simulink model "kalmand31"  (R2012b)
settings: Solver=ode4  StartTime=0.0  StopTime=10.0  RelTol=1e-3
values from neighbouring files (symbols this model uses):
  ampl = 2    [kalman_d2.m]    (also in kalman_d3.m; kalman_d4.m; diff_filter_1.m = 1)
  fanreg = 0.1    [kalman_d2.m]    (also in kalman_d3.m; kalman_d4.m)
  Kest = kalman(P,1,0.01),    [LQG_1.m]    (also in ss_zwei_eing_1.m = kalman(sys2, Q, R))
  my_sys11 = ss(my_sys11.a,my_sys11.b,eye(2,2),[0;0])    [kalman_d2.m]    (also in kalman_d3.m = ss(my_sys3.a, my_sys3.b(:,1), eye(2,2), 0); kalman_pegel_1.m = c2d(my_sys1,Ts,'zoh'))
  my_sys3 = c2d(my_sys2, Ts, 'zoh')    [kalman_d2.m]    (also in kalman_d3.m)
  Ts = 0.001    [fuellstnd_3.m]    (also in fuellstnd_31.m; kalman_d1.m = 0.05; kalman_d2.m = 0.1; kalman_d3.m = 0.1)
  vnd = 1e-4    (= 0.0001)    [kalman_1.m]    (also in kalman_10.m; kalman_11.m; kalman_12.m; kalman_13.m = 0.01)
  vny = 1e-6    (= 1e-06)    [kalman_1.m]    (also in kalman_10.m; kalman_11.m = ', num2str(vny),' )']); kalman_12.m = ', num2str(vny),' )']); kalman_13.m = ', num2str(vny),' )']))
libraries: simulink x2

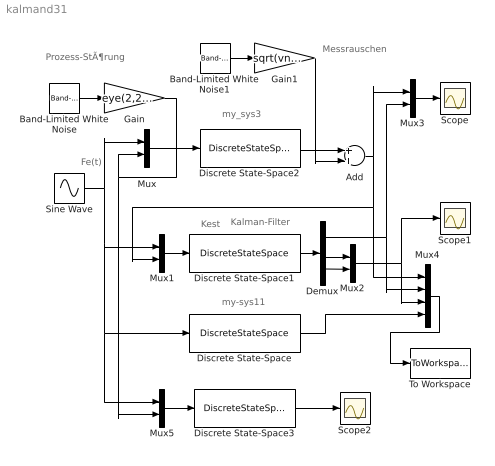
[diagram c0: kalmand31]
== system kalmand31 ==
  note: Fe(t)
  note: Prozess-StÃ¶rung
  note: Messrauschen
  note: Kalman-Filter
  note: my-sys11
  note: my_sys3
  note: Kest
  Add : Sum
  Band-Limited White Noise : simulink/Sources/Band-Limited White Noise  Cov=[Ts, Ts]  Ts=Ts  seed=[23341, 1965]
  Band-Limited White Noise1 : simulink/Sources/Band-Limited White Noise  Cov=[Ts]  Ts=Ts  seed=[267185]
  Demux : Demux  Outputs=3
  Discrete State-Space : DiscreteStateSpace  A=my_sys11.a  B=my_sys11.b  C=my_sys11.c  D=my_sys11.d  SampleTime=Ts
  Discrete State-Space1 : DiscreteStateSpace  A=Kest.a  B=Kest.b  C=Kest.c  D=Kest.d  SampleTime=Ts
  Discrete State-Space2 : DiscreteStateSpace  A=my_sys3.a  B=my_sys3.b  C=my_sys3.c  D=my_sys3.d  SampleTime=Ts
  Discrete State-Space3 : DiscreteStateSpace  A=my_sys3.a  B=my_sys3.b  C=eye(2,2)  D=[0,0,0;0,0,0]  SampleTime=Ts
  Gain : Gain  Gain=eye(2,2)*sqrt(vnd)  Multiplication=Matrix(K*u)
  Gain1 : Gain  Gain=sqrt(vny)
  Mux{,1..3,5} (5 alike) : Mux  Inputs=2
  Mux4 : Mux
  Scope : Scope
  Scope1 : Scope
  Scope2 : Scope
  Sine Wave : Sin  Amplitude=ampl  Frequency=2*pi*fanreg  SampleTime=Ts
  To Workspace : ToWorkspace  VariableName=y  SampleTime=-1  SaveFormat=Structure With Time
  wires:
  Band-Limited White Noise/1 -> Gain/1
  Mux/1 -> Discrete State-Space2/1
  Sine Wave/1 -> Mux/1, Mux5/1, Discrete State-Space/1, Mux1/1
  Mux1/1 -> Discrete State-Space1/1
  Band-Limited White Noise1/1 -> Gain1/1
  Discrete State-Space2/1 -> Add/1
  Gain1/1 -> Add/2
  Discrete State-Space1/1 -> Demux/1
  Demux/2 -> Mux2/1
  Demux/3 -> Mux2/2
  Demux/1 -> Mux3/2, Mux4/2
  Mux3/1 -> Scope/1
  Mux2/1 -> Mux4/3, Scope1/1
  Gain/1 -> Mux5/2, Mux/2
  Add/1 -> Mux3/1, Mux4/1, Mux1/2
  Discrete State-Space/1 -> Mux4/4
  Mux4/1 -> To Workspace/1
  Mux5/1 -> Discrete State-Space3/1
  Discrete State-Space3/1 -> Scope2/1
